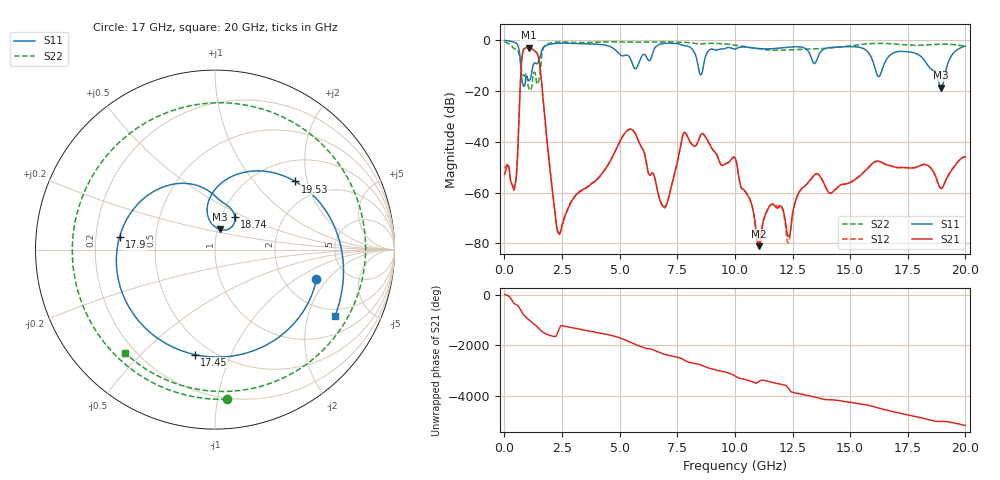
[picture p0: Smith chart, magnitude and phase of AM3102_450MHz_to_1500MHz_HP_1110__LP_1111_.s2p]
!Agilent Technologies,E8364B,MY43040894,A.07.50.67
!Agilent E8364B: A.07.50.67
!Date: Thursday, January 11, 2018 06:47:57
!Correction: S11(Full 2 Port(1,2))
!S21(Full 2 Port(1,2))
!S12(Full 2 Port(1,2))
!S22(Full 2 Port(1,2))
!S2P File: Measurements: S11, S21, S12, S22:
# Hz S  dB  R 50
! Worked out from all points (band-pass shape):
!   1601 points, 10 MHz to 20 GHz, reference 50 ohm
!   highest |S21| = -2.91 dB at 1.047 GHz (marker M1); lowest = -81.1 dB at 11.04 GHz (marker M2)
!   |S21| within 3 dB of the highest: 775.6 MHz to 1.45 GHz (674.6 MHz wide, 60.6 % of centre)
!   lowest |S11| = -18.7 dB at 18.95 GHz (marker M3), VSWR 1.26, Z = 51.7 + j11.7 ohm
!   |S11| at or under -10 dB: 705.2 MHz to 1.243 GHz (538.1 MHz wide, 55.2 % of centre); 16.05 GHz to 16.45 GHz (400.9 MHz wide, 2.47 % of centre); 18.38 GHz to 19.21 GHz (830.6 MHz wide, 4.42 % of centre)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
!   |S22| runs from -19.7 to -0.6 dB; largest |S21 - S12| = 0.00076
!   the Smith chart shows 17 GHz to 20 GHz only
!   S11 on the Smith chart (normalised r, x): 17 GHz: 3.02, -1.53; 17.45 GHz: 0.41, -0.74; 17.9 GHz: 0.30, +0.06; 18.74 GHz: 1.16, +0.44; 19.53 GHz: 1.46, +1.69; 20 GHz: 1.69, -3.01
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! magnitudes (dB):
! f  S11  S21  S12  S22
! 10 MHz  -0.1  -52.8  -50.5  -0.6
! 459.8 MHz  -0.9  -57.1  -56.8  -3.4
! 772.1 MHz  -16.1  -6.1  -6.1  -12.8
! 1.047 GHz  -15.8  -2.9  -2.9  -18.6
! 1.509 GHz  -7.7  -8.3  -8.4  -15.2
! 2.334 GHz  -1.2  -75.6  -75.6  -0.7
! 3.346 GHz  -1.4  -59.2  -59.2  -0.9
! 5.47 GHz  -7.3  -35.0  -35.0  -0.8
! 6.682 GHz  -1.8  -60.7  -60.8  -0.7
! 7.819 GHz  -2.2  -36.3  -36.2  -0.9
! 10.01 GHz  -3.4  -46.3  -46.3  -2.0
! 11.04 GHz  -3.3  -81.1  -80.0  -3.4
! 12.33 GHz  -2.7  -77.2  -79.5  -3.8
! 13.34 GHz  -7.5  -54.2  -54.3  -3.4
! 16.68 GHz  -6.4  -49.3  -49.3  -1.3
! 17 GHz  -4.6  -50.0  -50.1  -1.6
! 17.45 GHz  -4.5  -50.2  -50.1  -1.9
! 17.9 GHz  -5.4  -49.8  -49.8  -2.0
! 18.74 GHz  -13.4  -54.3  -54.3  -1.6
! 18.95 GHz  -18.7  -58.4  -58.3  -1.5
! 19.53 GHz  -4.6  -49.7  -49.6  -1.8
! 20 GHz  -2.3  -45.8  -46.0  -2.3
